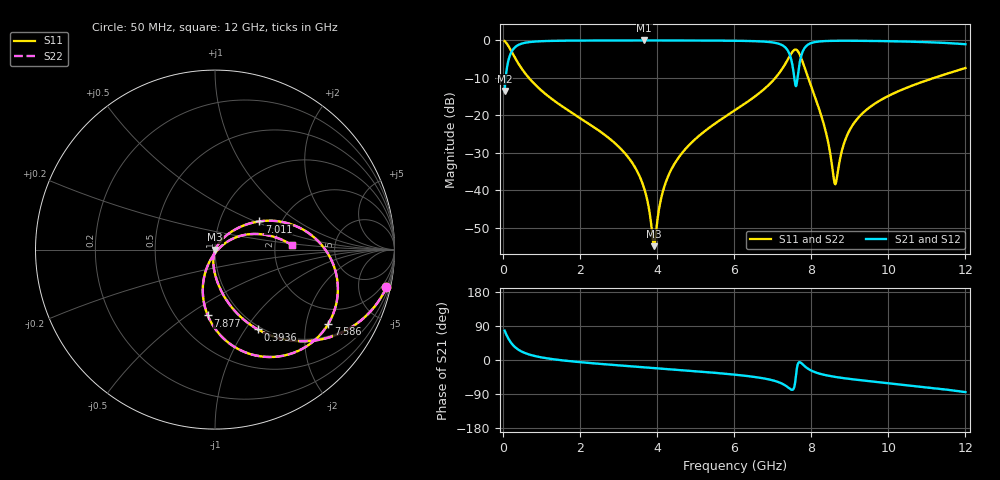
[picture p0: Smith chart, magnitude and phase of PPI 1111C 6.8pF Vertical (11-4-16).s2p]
# GHz S MA R 50
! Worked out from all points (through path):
!   1601 points, 50 MHz to 12 GHz, reference 50 ohm
!   highest |S21| = -0.02 dB at 3.672 GHz (marker M1); lowest = -13.5 dB at 50 MHz (marker M2)
!   group delay of S21, straight-line fit = 22 ps
!   lowest |S11| = -54.8 dB at 3.926 GHz (marker M3), VSWR 1.00, Z = 50.2 - j0.0646 ohm
!   |S11| at or under -10 dB: 680.2 MHz to 7.071 GHz (6.391 GHz wide, 165 % of centre); 7.923 GHz to 11.19 GHz (3.263 GHz wide, 34.2 % of centre)
!   |S22| runs from -54.8 to -0.2 dB; largest |S21 - S12| = 0
!   S11 on the Smith chart (normalised r, x): 50 MHz: 0.96, -9.06; 393.6 MHz: 0.96, -1.14; 7.011 GHz: 1.54, +0.53; 7.586 GHz: 1.40, -2.69; 7.877 GHz: 0.71, -0.60; 12 GHz: 2.49, +0.16
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0.05  0.9775 -12.5  0.211 77.5  0.211 77.5  0.9775 -12.5
0.1844375  0.7817 -39.6  0.6233 50.4  0.6233 50.4  0.7817 -39.6
0.3935625  0.5044 -61.8  0.8629 28.1  0.8629 28.1  0.5044 -61.8
2.044156  0.08973 -95.2  0.9946 -6.0  0.9946 -6.0  0.08973 -95.2
3.142063  0.03251 -102.5  0.9977 -15.2  0.9977 -15.2  0.03251 -102.5
3.672344  0.01055 -99.9  0.998 -19.3  0.998 -19.3  0.01055 -99.9
3.926281  0.001812 -20.8  0.998 -21.2  0.998 -21.2  0.001812 -20.8
4.038312  0.005015 46.2  0.9979 -22.1  0.9979 -22.1  0.005015 46.2
4.239969  0.01331 58.0  0.9977 -23.6  0.9977 -23.6  0.01331 58.0
4.591  0.02876 59.4  0.9972 -26.3  0.9972 -26.3  0.02876 59.4
6.025  0.1176 49.3  0.9887 -38.7  0.9887 -38.7  0.1176 49.3
7.010875  0.2918 32.6  0.9377 -53.8  0.9377 -53.8  0.2918 32.6
7.376844  0.536 9.3  0.7543 -70.5  0.7543 -70.5  0.536 9.3
7.585969  0.7549 -33.3  0.2629 -58.2  0.2629 -58.2  0.7549 -33.3
7.698  0.658 -65.2  0.4897 -5.6  0.4897 -5.6  0.658 -65.2
7.87725  0.369 -96.3  0.8454 -20.0  0.8454 -20.0  0.369 -96.3
8.019156  0.229 -107.3  0.9287 -28.7  0.9287 -28.7  0.229 -107.3
8.362719  0.06561 -113.9  0.9797 -39.7  0.9797 -39.7  0.06561 -113.9
8.624125  0.01211 -40.7  0.9875 -44.6  0.9875 -44.6  0.01211 -40.7
9.064781  0.07285 32.6  0.9885 -50.7  0.9885 -50.7  0.07285 32.6
10.01331  0.1832 26.5  0.9758 -61.4  0.9758 -61.4  0.1832 26.5
12  0.4289 3.4  0.8885 -84.7  0.8885 -84.7  0.4289 3.4
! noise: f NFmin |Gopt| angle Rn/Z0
0.05  0.0003942  0.8838  2.502  0.0007355
1.372  0.003654  0.6671  8.242  0.002096
2.701  0.006065  0.62  15.05  0.002928
4.031  0.008471  0.6046  21.73  0.003826
5.36  0.01175  0.6249  28.19  0.005532
6.682  0.02291  0.7491  34.76  0.01678
8.012  0.05795  0.8764  41.8  0.08848
9.341  0.02416  0.6984  47.42  0.01321
10.67  0.02547  0.6884  52.62  0.01287
12  0.0381  0.7655  58.29  0.02534
